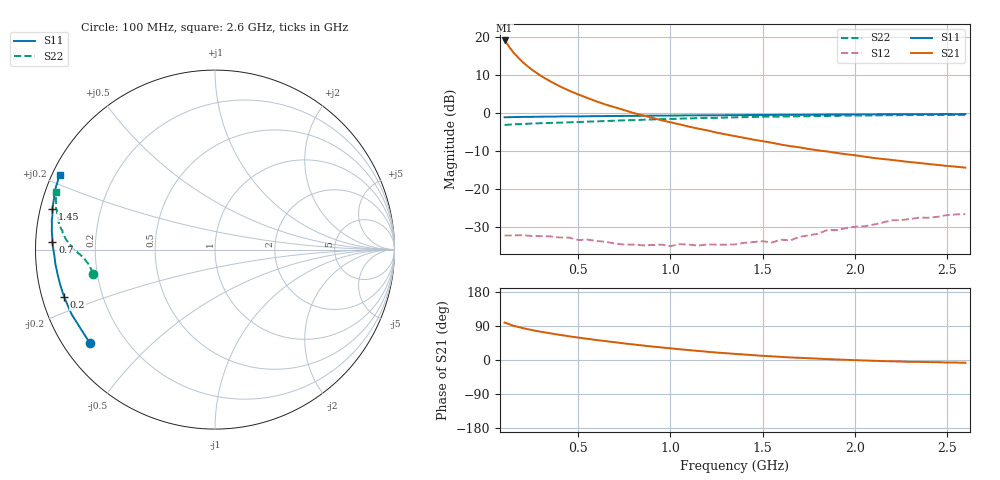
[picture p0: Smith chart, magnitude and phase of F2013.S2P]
!  POLYFET RF DEVICES
!  F2013
!  S PARAMETERS
!  VDS=28V, IDQ=800mA
! Date: Mon Aug  5 14:20:22 1991
# MHZ S MA R 50
! Bias (V mA) : V1=2.8989000  I1=0.0110650  V2=27.999120  I2=799.60300
!  FREQ  S11  S11 ANG  S21  S21 ANG  S12  S12 ANG  S22  S22 ANG!
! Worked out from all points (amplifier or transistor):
!   51 points, 100 MHz to 2.6 GHz, reference 50 ohm
!   highest |S21| = 19.0 dB at 100 MHz (marker M1)
!   |S21| within 3 dB of that: start of sweep to 145.1 MHz
!   unconditionally stable (mu >= 1): 633.9 MHz to 1.937 GHz
!   at 500 MHz: K = 0.79, MSG = 19.1 dB, |S12| = -33.5 dB
!   at 1.35 GHz: K = 1.63, MAG = 9.6 dB, |S12| = -34.6 dB
!   at 2.6 GHz: K = 0.56, MSG = 6.1 dB, |S12| = -26.7 dB
!   S11 on the Smith chart (normalised r, x): 100 MHz: 0.08, -0.33; 200 MHz: 0.06, -0.15; 700 MHz: 0.05, +0.02; 1.45 GHz: 0.03, +0.12; 2.6 GHz: 0.02, +0.23
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100  0.8703 -143.3  8.923 98.7  0.02428 15.1  0.691 -168.8
150  0.8766 -155.7  6.086 90.1  0.02432 8.3  0.7042 -172.2
200  0.8809 -162.5  4.585 84.0  0.02453 5.1  0.7107 -173.6
250  0.8842 -167.0  3.651 78.8  0.02389 5.4  0.722 -175.1
300  0.8869 -170.1  3.018 74.2  0.0238 4.0  0.7284 -175.9
350  0.8894 -172.6  2.57 70.1  0.02362 2.2  0.7346 -176.5
400  0.8926 -174.6  2.225 66.3  0.02284 0.8  0.7406 -177.0
450  0.8941 -176.3  1.95 62.6  0.0228 2.1  0.7474 -177.5
550  0.8986 -179.2  1.561 55.9  0.02141 1.3  0.763 -178.6
600  0.9018 179.6  1.405 52.6  0.02055 2.5  0.7698 -179.1
700  0.9064 177.5  1.176 46.7  0.01897 4.7  0.7873 180.0
800  0.9097 175.5  0.9909 41.0  0.01845 9.9  0.7986 178.6
950  0.916 172.9  0.7977 33.2  0.01844 14.5  0.8219 176.9
1100  0.9215 170.5  0.6566 26.1  0.01839 21.8  0.8423 174.9
1350  0.929 167.0  0.4925 16.1  0.01852 37.9  0.8696 171.8
1450  0.9341 165.8  0.4429 12.8  0.01992 39.0  0.8791 170.5
1650  0.9385 163.4  0.3638 6.8  0.02094 50.0  0.8944 168.3
1800  0.943 161.9  0.3203 3.6  0.02557 53.3  0.9057 166.7
1850  0.9456 161.3  0.3093 2.4  0.02859 55.8  0.9062 166.3
2050  0.9495 159.4  0.2654 -1.3  0.03208 55.0  0.9191 164.5
2200  0.9536 158.0  0.2396 -3.5  0.03857 56.4  0.9261 163.2
2600  0.9597 154.3  0.1896 -7.2  0.04638 53.5  0.9402 160.0
